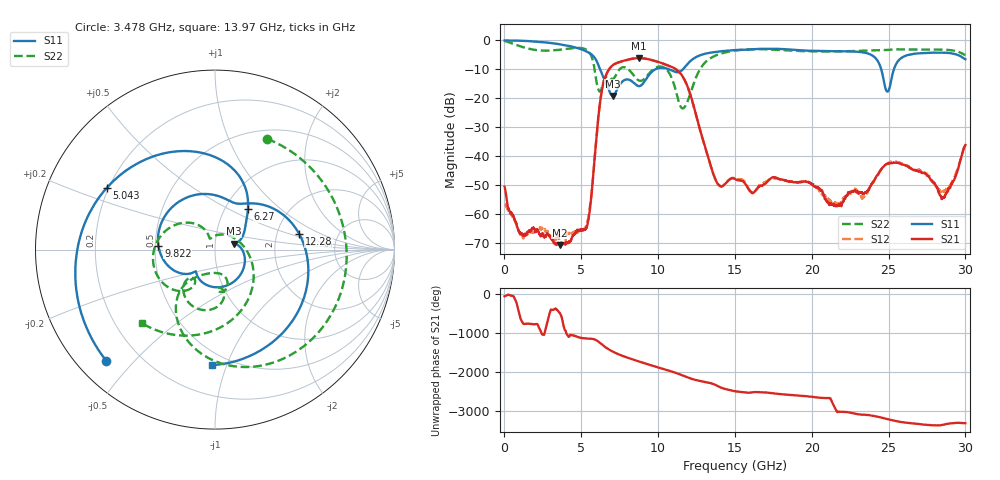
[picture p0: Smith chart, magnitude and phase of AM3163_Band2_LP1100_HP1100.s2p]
!Agilent Technologies,E8364B,MY43040894,A.07.50.67
!Agilent E8364B: A.07.50.67
!Date: Thursday, August 20, 2020 11:14:02
!Correction: S11(Full 2 Port(1,2))
!S21(Full 2 Port(1,2))
!S12(Full 2 Port(1,2))
!S22(Full 2 Port(1,2))
!S2P File: Measurements: S11, S21, S12, S22:
# Hz S  dB  R 50
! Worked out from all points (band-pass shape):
!   3201 points, 10 MHz to 30 GHz, reference 50 ohm
!   highest |S21| = -6.15 dB at 8.763 GHz (marker M1); lowest = -70.7 dB at 3.609 GHz (marker M2)
!   |S21| within 3 dB of the highest: 6.933 GHz to 10.88 GHz (3.948 GHz wide, 44.3 % of centre)
!   lowest |S11| = -19.2 dB at 7.039 GHz (marker M3), VSWR 1.25, Z = 61.5 + j4.07 ohm
!   |S11| at or under -10 dB: 6.217 GHz to 9.821 GHz (3.604 GHz wide, 44.9 % of centre); 10.71 GHz to 11.62 GHz (907.6 MHz wide, 8.13 % of centre); 24.52 GHz to 25.35 GHz (825.3 MHz wide, 3.31 % of centre)
!   |S22| runs from -23.5 to -0.2 dB; largest |S21 - S12| = 0.0037
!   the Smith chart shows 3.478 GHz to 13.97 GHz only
!   S11 on the Smith chart (normalised r, x): 3.478 GHz: 0.08, -0.42; 5.043 GHz: 0.19, +0.26; 6.27 GHz: 1.28, +0.63; 9.822 GHz: 0.52, +0.03; 12.28 GHz: 2.68, +0.59; 13.97 GHz: 0.40, -0.89
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1e7  -0.03 -2.5  -50.58 -56.3  -56.71 -73.8  -0.21 -8.2
7.5975e8  -0.10 -28.6  -63.15 163.9  -63.25 -55.1  -1.57 -83.3
1.65945e9  -0.27 -62.7  -65.99 -43.8  -65.71 -86.3  -2.98 -163.8
3.477594e9  -1.24 -134.2  -70.21 -66.4  -67.95 -134.9  -3.31 64.8
3.6088e9  -1.35 -139.7  -70.73 -125.8  -70.56 61.4  -3.24 56.1
5.014581e9  -3.11 152.0  -65.56 -42.6  -65.72 -42.2  -2.67 -42.4
5.042697e9  -3.17 150.3  -65.80 -47.7  -65.81 -48.6  -2.69 -44.7
6.270412e9  -10.73 50.9  -19.61 171.2  -19.67 170.9  -17.46 -81.0
7.038906e9  -19.21 17.3  -8.63 -35.0  -8.67 -35.1  -13.39 -82.9
7.919862e9  -13.54 -70.4  -6.82 179.7  -6.87 179.9  -9.50 -113.7
8.763331e9  -15.83 -131.2  -6.15 67.6  -6.16 67.7  -13.90 -129.2
9.822353e9  -10.00 175.9  -7.17 -61.0  -7.20 -61.2  -9.50 -141.3
1.000979e10  -9.61 159.8  -7.47 -82.9  -7.52 -83.0  -9.10 -152.8
1.227778e10  -6.41 10.2  -21.96 -28.3  -22.07 -27.7  -15.59 3.5
1.397409e10  -3.83 -91.5  -50.17 138.6  -50.18 141.4  -4.76 -134.8
1.5005e10  -3.36 -136.6  -47.94 24.5  -47.72 27.2  -3.55 179.0
1.782593e10  -2.94 97.2  -47.84 -45.8  -47.92 -47.2  -3.29 60.3
2.000958e10  -3.62 -13.3  -49.75 -116.7  -49.80 -118.7  -3.83 -28.0
2.349592e10  -4.32 -149.5  -52.76 138.1  -53.73 135.4  -3.55 -133.5
2.500479e10  -17.31 -150.0  -42.53 20.1  -42.37 22.4  -3.29 -171.0
2.854736e10  -4.25 105.0  -54.30 -116.4  -52.32 -110.7  -3.23 96.6
3e10  -6.53 50.0  -36.20 -78.8  -36.16 -80.2  -5.07 53.3
